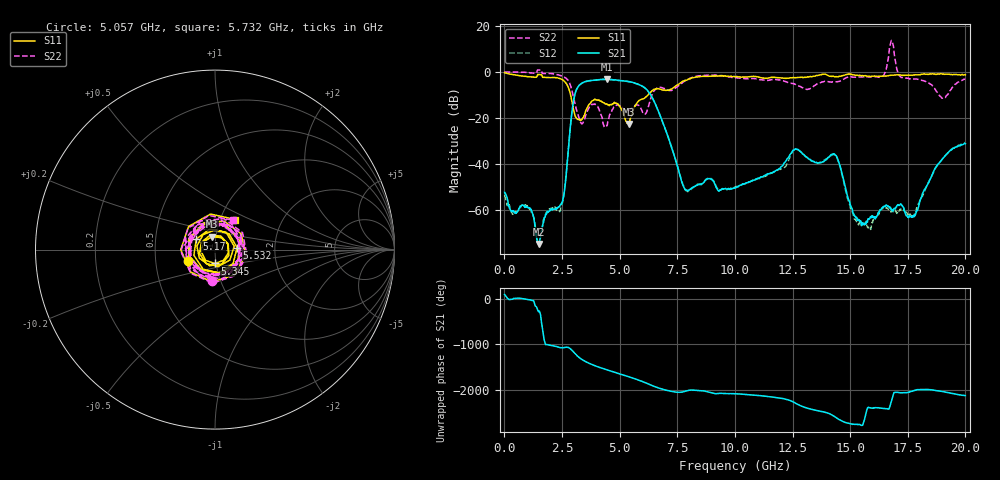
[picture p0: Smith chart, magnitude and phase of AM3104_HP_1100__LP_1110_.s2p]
!Created with skrf (http://scikit-rf.org).
# Hz S RI R 50.0
!freq ReS11 ImS11 ReS21 ImS21 ReS12 ImS12 ReS22 ImS22
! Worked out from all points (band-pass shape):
!   1601 points, 10 MHz to 20 GHz, reference 50 ohm
!   highest |S21| = -3.26 dB at 4.458 GHz (marker M1); lowest = -74.6 dB at 1.497 GHz (marker M2)
!   |S21| within 3 dB of the highest: 3.215 GHz to 5.988 GHz (2.774 GHz wide, 60.3 % of centre)
!   lowest |S11| = -22.6 dB at 5.395 GHz (marker M3), VSWR 1.16, Z = 47.9 + j6.98 ohm
!   |S11| at or under -10 dB: 2.872 GHz to 6.23 GHz (3.358 GHz wide, 73.8 % of centre)
!   |S22| runs from -24.0 to 13.6 dB; largest |S21 - S12| = 0.077
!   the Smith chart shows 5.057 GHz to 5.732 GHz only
!   S11 on the Smith chart (normalised r, x): 5.057 GHz: 0.74, -0.10; 5.17 GHz: 0.81, +0.10; 5.345 GHz: 0.99, -0.15; 5.532 GHz: 1.28, +0.03; 5.732 GHz: 1.18, +0.41
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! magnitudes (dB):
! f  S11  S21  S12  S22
! 10 MHz  -0.4  -52.2  -53.3  -0.1
! 1.059 GHz  -2.2  -59.1  -59.1  -0.4
! 1.497 GHz  -1.2  -74.6  -75.3  0.8
! 2.496 GHz  -3.3  -56.7  -57.5  -1.9
! 2.996 GHz  -16.3  -12.8  -12.8  -10.9
! 3.346 GHz  -20.8  -5.0  -5.1  -22.5
! 4.458 GHz  -14.0  -3.3  -3.3  -23.3
! 5.057 GHz  -15.8  -3.8  -3.9  -15.1
! 5.17 GHz  -18.4  -3.9  -3.9  -16.2
! 5.345 GHz  -22.2  -4.1  -4.2  -16.9
! 5.395 GHz  -22.6  -4.2  -4.3  -16.8
! 5.532 GHz  -18.1  -4.5  -4.5  -15.7
! 5.732 GHz  -13.9  -5.1  -5.2  -14.3
! 6.682 GHz  -7.3  -17.1  -17.1  -6.8
! 7.881 GHz  -3.7  -51.2  -51.5  -3.7
! 10.01 GHz  -2.2  -50.4  -50.1  -2.7
! 13.34 GHz  -2.2  -38.6  -38.6  -6.8
! 14.37 GHz  -2.1  -36.1  -36.4  -4.4
! 15.51 GHz  -1.6  -66.1  -66.1  -2.2
! 16.68 GHz  -1.6  -58.4  -60.2  7.2
! 17.76 GHz  -1.4  -62.4  -61.9  -3.1
! 20 GHz  -1.3  -31.1  -30.7  -3.2
